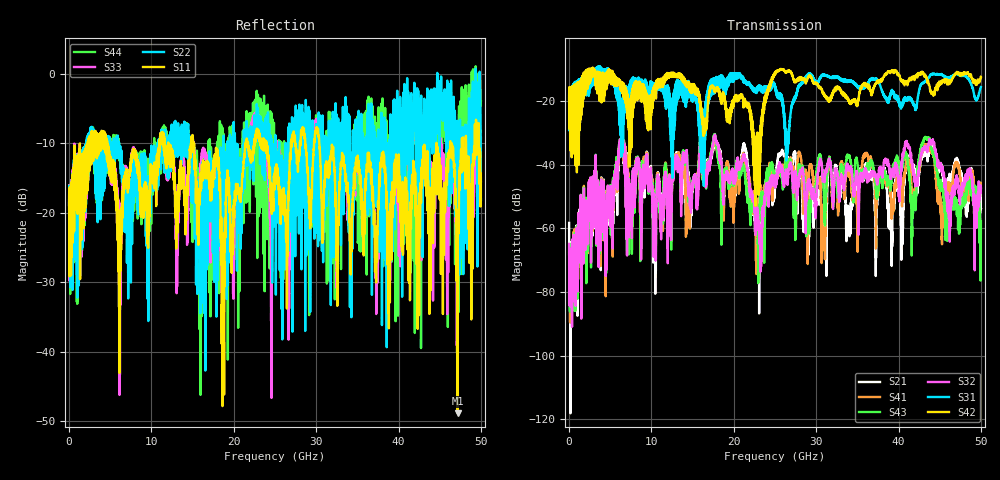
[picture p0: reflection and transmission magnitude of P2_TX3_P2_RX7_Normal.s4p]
!Keysight Technologies,N5225B,MY57041031,A.13.20.10
!Date: Friday, May 31, 2019 11:37:42
!Correction: S11(Full 4 Port(1,2,3,4))
!S12(Full 4 Port(1,2,3,4))
!S13(Full 4 Port(1,2,3,4))
!S14(Full 4 Port(1,2,3,4))
!S21(Full 4 Port(1,2,3,4))
!S22(Full 4 Port(1,2,3,4))
!S23(Full 4 Port(1,2,3,4))
!S24(Full 4 Port(1,2,3,4))
!S31(Full 4 Port(1,2,3,4))
!S32(Full 4 Port(1,2,3,4))
!S33(Full 4 Port(1,2,3,4))
!S34(Full 4 Port(1,2,3,4))
!S41(Full 4 Port(1,2,3,4))
!S42(Full 4 Port(1,2,3,4))
!S43(Full 4 Port(1,2,3,4))
!S44(Full 4 Port(1,2,3,4))
!S4P File: Measurements: <S11,S12,S13,S14>,
!<S21,S22,S23,S24>,
!<S31,S32,S33,S34>,
!<S41,S42,S43,S44>:
# Hz S  dB  R 50.0
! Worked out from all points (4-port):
!   5000 points, 10 MHz to 50 GHz, reference 50 ohm
!   strongest paths, dB at 10 MHz, 12.51 GHz, 25.01 GHz, 37.51 GHz, 50 GHz:
!     S42: -19.4, -12.1, -11.6, -13.6, -12.4
!     S31: -19.5, -42.6, -16.1, -13.6, -15.6
!     S32: -64.9, -43.6, -44.5, -44.2, -47.4
!     S43: -83.5, -46.6, -45.4, -47.6, -57.7
!     S41: -67.6, -46.0, -43.4, -48.0, -47.4
!     S21: -58.3, -43.1, -46.5, -45.5, -53.8
!   lowest |S11| = -48.9 dB at 47.18 GHz (marker M1), VSWR 1.01, Z = 49.9 - j0.333 ohm
!   |S11| at or under -10 dB: 4.63 GHz to 10.95 GHz (6.317 GHz wide, 81.1 % of centre); 15.14 GHz to 21.46 GHz (6.324 GHz wide, 34.6 % of centre); 30.38 GHz to 44.61 GHz (14.23 GHz wide, 37.9 % of centre)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
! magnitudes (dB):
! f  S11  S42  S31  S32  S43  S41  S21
! 10 MHz  -19.6  -19.4  -19.5  -64.9  -83.5  -67.6  -58.3
! 6.32 GHz  -25.4  -14.1  -22.6  -32.8  -32.4  -33.1  -33.7
! 21.3 GHz  -12.1  -19.3  -13.4  -37.3  -41.9  -38.2  -33.7
! 23.21 GHz  -9.8  -28.7  -16.6  -63.5  -52.5  -47.8  -53.7
! 43.41 GHz  -15.7  -12.8  -13.3  -35.0  -31.7  -33.8  -36.6
! 47.18 GHz  -48.9  -11.3  -11.4  -44.6  -55.8  -40.7  -38.7
! 50 GHz  -15.5  -12.4  -15.6  -47.4  -57.7  -47.4  -53.8
